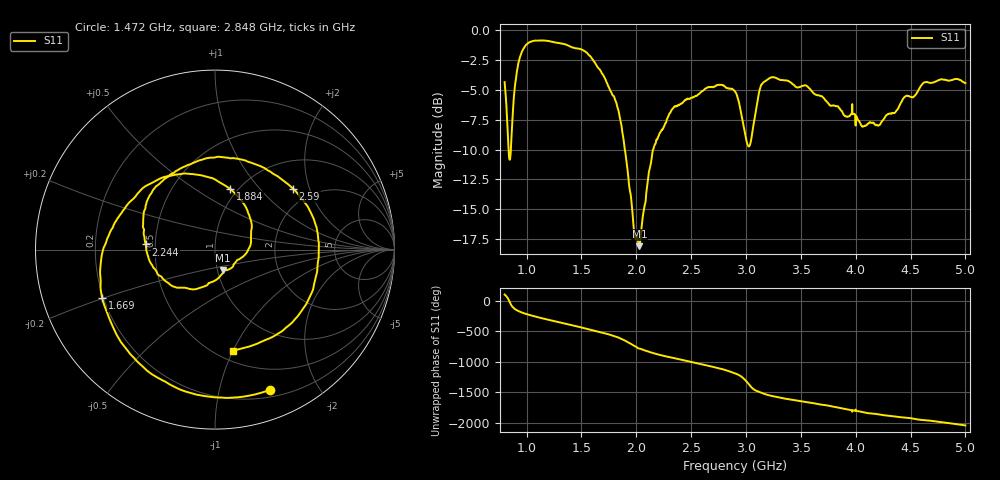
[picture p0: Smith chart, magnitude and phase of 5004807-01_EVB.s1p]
#  HZ  S  RI  R  50.00
! Rohde & Schwarz ZVA/B
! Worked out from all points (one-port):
!   1601 points, 800 MHz to 5 GHz, reference 50 ohm
!   lowest |S11| = -18.1 dB at 2.029 GHz (marker M1), VSWR 1.28, Z = 53.3 - j12.5 ohm
!   |S11| at or under -10 dB: 835.8 MHz to 857.1 MHz (21.26 MHz wide, 2.51 % of centre); 1.896 GHz to 2.153 GHz (256.7 MHz wide, 12.7 % of centre)
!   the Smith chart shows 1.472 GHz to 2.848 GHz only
!   S11 on the Smith chart (normalised r, x): 1.472 GHz: 0.27, -1.43; 1.669 GHz: 0.19, -0.20; 1.884 GHz: 0.92, +0.71; 2.244 GHz: 0.44, +0.03; 2.59 GHz: 1.60, +1.56; 2.848 GHz: 0.60, -1.00
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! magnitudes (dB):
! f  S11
! 800 MHz  -4.3
! 834.1 MHz  -9.8
! 847.2 MHz  -10.8
! 907.6 MHz  -3.8
! 968 MHz  -1.6
! 1.07 GHz  -0.9
! 1.325 GHz  -1.1
! 1.472 GHz  -1.5
! 1.669 GHz  -3.3
! 1.85 GHz  -7.3
! 1.884 GHz  -9.1
! 1.981 GHz  -17.1
! 2.029 GHz  -18.1
! 2.147 GHz  -10.3
! 2.244 GHz  -8.3
! 2.375 GHz  -6.3
! 2.59 GHz  -5.2
! 2.848 GHz  -4.9
! 2.9 GHz  -5.1
! 3.026 GHz  -9.7
! 3.152 GHz  -4.4
! 3.425 GHz  -4.5
! 3.95 GHz  -7.1
! 4.066 GHz  -8.1
! 4.205 GHz  -8.0
! 4.475 GHz  -5.5
! 4.635 GHz  -4.3
! 5 GHz  -4.4
